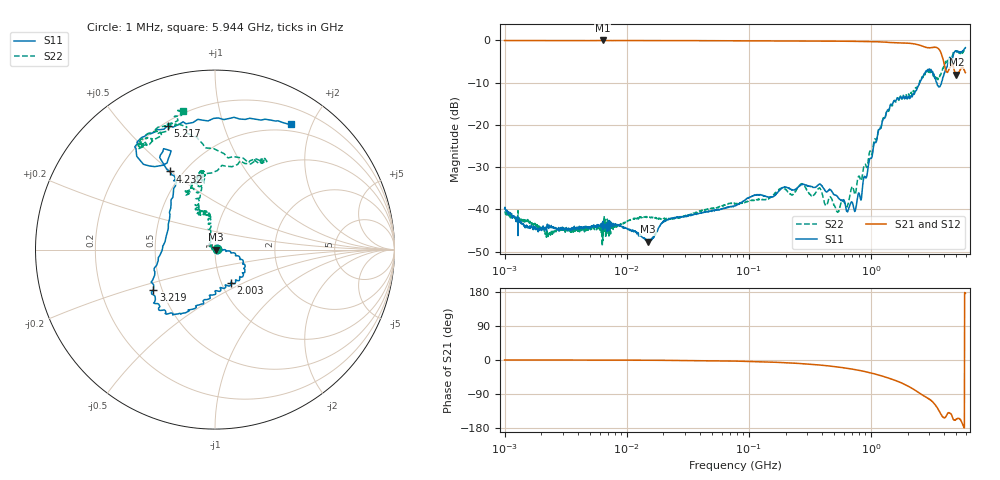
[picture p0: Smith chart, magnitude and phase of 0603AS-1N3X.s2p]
!s-Parameter Generated by FASTRON Sdn. Bhd.
!FASTRON P/N : 0603AS-1N3X
!Keysight Technologies: E5071C_MY46733604_B.14.02
!Date: Tue Nov 21 15:49:39 2023
!Version  :Rev01  Tue Nov 21 15:49:39 2023
!Data & Calibration Information:
!Freq  S11:SOLT2(ON)  S21:SOLT2(ON)  S12:SOLT2(ON)  S22:SOLT2(ON)
!PortZ  Port1:50+j0  Port2:50+j0
!When reading reference impedance value at option line is always used.
! Remarks : This data is being provided solely for informational purposes.
# Hz S dB R 50
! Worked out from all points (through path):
!   1599 points, 1 MHz to 5.944 GHz, reference 50 ohm
!   highest |S21| = -0.03 dB at 6.378 MHz (marker M1); lowest = -8.1 dB at 5.021 GHz (marker M2)
!   group delay of S21, straight-line fit = 91.5 ps
!   lowest |S11| = -47.6 dB at 14.93 MHz (marker M3), VSWR 1.01, Z = 50.4 - j0.0579 ohm
!   |S11| at or under -10 dB: start of sweep to 2.518 GHz; 3.468 GHz to 3.783 GHz (315.4 MHz wide, 8.7 % of centre)
!   |S22| runs from -48.7 to -1.9 dB; largest |S21 - S12| = 0.014
!   S11 on the Smith chart (normalised r, x): 1 MHz: 1.02, +0.00; 2.003 GHz: 1.10, -0.43; 3.219 GHz: 0.45, -0.24; 4.232 GHz: 0.43, +0.50; 5.217 GHz: 0.22, +0.66; 5.944 GHz: 0.40, +1.70
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1000000  -39.80 13.5  -0.05 0.0  -0.07 0.1  -40.50 17.5
1528420  -44.10 -0.5  -0.06 -0.0  -0.07 0.0  -42.40 -11.0
2215059  -44.10 19.6  -0.06 -0.1  -0.07 -0.1  -45.50 22.3
4277066  -44.50 10.2  -0.06 -0.2  -0.07 -0.2  -45.00 12.9
6378092  -44.80 19.9  -0.03 -0.3  -0.06 -0.3  -47.40 -6.6
1.493236e7  -47.60 -7.9  -0.06 -0.6  -0.07 -0.6  -41.70 9.9
1.81383e7  -44.50 11.8  -0.06 -0.8  -0.08 -0.7  -42.30 19.3
7.715586e7  -39.20 35.6  -0.08 -2.9  -0.10 -2.9  -38.70 36.2
2.706977e8  -34.10 46.5  -0.14 -9.6  -0.15 -9.6  -34.00 58.1
3.28998e8  -34.60 33.5  -0.16 -11.5  -0.17 -11.5  -36.80 66.7
3.795645e8  -34.00 43.2  -0.17 -13.2  -0.18 -13.3  -35.00 74.0
5.345736e8  -37.00 18.1  -0.20 -18.4  -0.21 -18.4  -40.70 111.0
7.407998e8  -40.40 0.8  -0.25 -25.4  -0.25 -25.4  -36.50 159.0
1.399393e9  -16.40 -21.5  -0.48 -47.9  -0.49 -48.0  -16.80 102.0
2.003084e9  -13.70 -65.0  -0.67 -68.4  -0.69 -68.5  -13.60 108.0
2.804647e9  -7.43 -122.0  -1.67 -97.5  -1.68 -97.4  -7.51 98.4
3.219478e9  -7.77 -147.0  -1.68 -111.0  -1.67 -111.0  -7.94 107.0
3.705459e9  -10.70 153.0  -2.59 -140.0  -2.59 -140.0  -8.18 109.0
4.231938e9  -5.97 120.0  -7.60 -142.0  -7.61 -142.0  -4.88 59.5
5.020705e9  -2.57 121.0  -8.12 -156.0  -8.14 -156.0  -2.58 118.0
5.216564e9  -2.64 111.0  -7.76 -154.0  -7.78 -154.0  -2.78 124.0
5.94404e9  -1.75 58.9  -7.66 176.0  -7.64 176.0  -2.02 103.0
